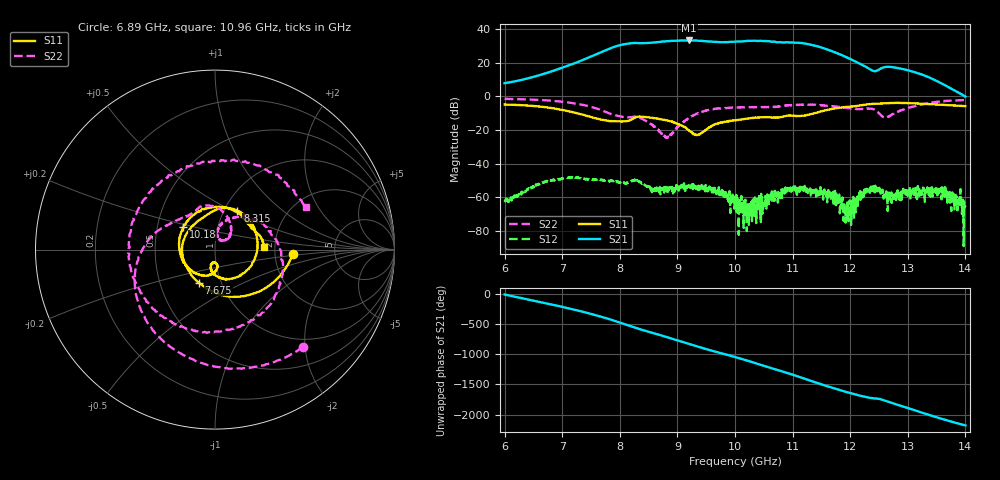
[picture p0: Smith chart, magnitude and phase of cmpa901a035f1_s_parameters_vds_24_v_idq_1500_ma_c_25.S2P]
!Keysight Technologies,E5071C,MY46110325,B.14.03
!Date: Wed Mar 10 11:00:59 2021
!Data & Calibration Information:
!Freq	S11:SOLT2(ON)	S21:SOLT2(ON)	S12:SOLT2(ON)	S22:SOLT2(ON)
!PortZ  Port1:50+j0  Port2:50+j0
!Above PortZ is port z conversion or system Z0 setting when saving the data.
!When reading, reference impedance value at option line is always used.
# Hz S dB R 50
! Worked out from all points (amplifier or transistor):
!   1601 points, 6 GHz to 14 GHz, reference 50 ohm
!   highest |S21| = 33.3 dB at 9.205 GHz (marker M1)
!   |S21| within 3 dB of that: 7.978 GHz to 11.38 GHz (3.397 GHz wide, 35.1 % of centre)
!   unconditionally stable (mu >= 1): start of sweep to end of sweep
!   at 7.33 GHz: K = 7.05, MAG = 23.4 dB, |S12| = -48.4 dB
!   at 10 GHz: K = 11.44, MAG = 33.8 dB, |S12| = -62.2 dB
!   at 14 GHz: K = 277.68, MAG = 5.4 dB, |S12| = -65.8 dB
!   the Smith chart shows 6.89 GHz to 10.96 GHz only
!   S11 on the Smith chart (normalised r, x): 6.89 GHz: 2.51, -0.15; 7.675 GHz: 0.78, -0.30; 8.315 GHz: 1.15, +0.53; 10.18 GHz: 0.68, +0.18; 10.96 GHz: 1.74, +0.06
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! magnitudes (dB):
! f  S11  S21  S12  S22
! 6 GHz  -4.8  7.9  -62.7  -1.4
! 6.89 GHz  -7.3  15.8  -49.6  -2.7
! 7.335 GHz  -10.6  21.4  -48.7  -4.9
! 7.675 GHz  -13.8  26.3  -49.8  -8.1
! 8.315 GHz  -12.0  31.8  -50.2  -12.2
! 8.67 GHz  -13.3  32.4  -54.5  -20.2
! 8.835 GHz  -14.4  32.9  -56.4  -24.4
! 9.205 GHz  -20.3  33.3  -54.1  -12.5
! 9.36 GHz  -22.6  33.2  -55.6  -9.9
! 10 GHz  -14.2  32.6  -62.2  -6.6
! 10.18 GHz  -13.3  32.9  -64.2  -6.4
! 10.46 GHz  -12.4  33.1  -60.8  -6.3
! 10.96 GHz  -11.3  32.1  -55.0  -5.1
! 11.34 GHz  -10.4  30.6  -55.6  -4.8
! 11.72 GHz  -7.2  26.4  -60.3  -5.9
! 11.94 GHz  -6.2  23.4  -73.3  -6.8
! 12.04 GHz  -5.9  21.5  -67.7  -7.2
! 12.18 GHz  -5.3  19.4  -56.3  -7.4
! 12.32 GHz  -4.6  16.7  -56.0  -7.3
! 12.67 GHz  -3.9  17.6  -55.8  -12.0
! 13.63 GHz  -5.0  7.0  -56.6  -2.8
! 14 GHz  -5.7  0.0  -65.8  -2.1
